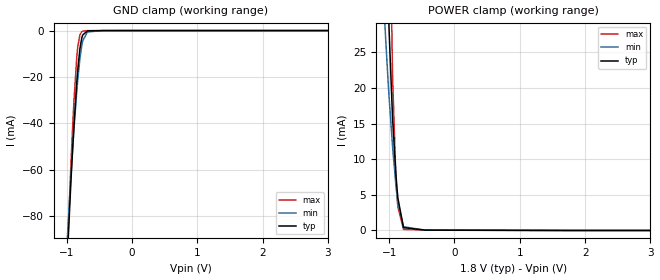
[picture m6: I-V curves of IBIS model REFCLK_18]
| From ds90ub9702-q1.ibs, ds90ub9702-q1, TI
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|   REFCLK_18 model
[Model]   REFCLK_18
Model_type   Input
Vinl = 0.63
Vinh = 1.17
|   typ   min   max
C_comp   1.10571pF   1.21238pF   5pF
[Voltage Range]   1.8   1.71   1.89
[Temperature Range]   27   105   -40
[Power Clamp Reference]   1.8   1.71   1.89
[GND Clamp Reference]   0   0   0
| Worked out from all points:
|   GND clamp passes 1 mA (typ) near -0.72 V on its own axis
|   POWER clamp passes 1 mA (typ) near -0.79 V on its own axis
[GND Clamp]
|   Voltage   I(typ)   I(min)   I(max)
-1.8V     -695.2mA   -622.8mA   -751.1mA
-1.001V   -105mA     -95.31mA   -104mA
-936mV    -66.2mA    -63.73mA   -59.18mA
-909mV    -51.71mA   -51.7mA    -42.45mA
-887.4mV  -40.99mA   -42.6mA    -30.38mA
-844.2mV  -22.35mA   -26.22mA   -11.45mA
-828mV    -16.57mA   -20.87mA   -6.784mA
-795.6mV  -7.686mA   -11.94mA   -1.813mA
-757.8mV  -2.294mA   -5.08mA    -324.2uA
-682.2mV  -140uA     -594.6uA   -25.34uA
-444.6mV  -9.322uA   -8.429uA   -11.13uA
3.6V      0A         0A         0A
[POWER Clamp]
|   Voltage   I(typ)   I(min)   I(max)
-1.8V     913.3mA    660mA      1.143A
-1.076V   62.45mA    31.29mA    126.5mA
-1.055V   49.98mA    27.29mA    103mA
-1.012V   31.67mA    20.38mA    61.71mA
-1.001V   28.28mA    18.81mA    53.01mA
-946.8mV  15.76mA    11.75mA    21.59mA
-898.2mV  8.22mA     6.549mA    7.96mA
-876.6mV  5.652mA    4.69mA     4.554mA
-865.8mV  4.556mA    3.885mA    3.297mA
-779.4mV  399.7uA    531uA      153.8uA
-444.6mV  47.04uA    39.07uA    58.46uA
3.6V      0A         0A         0A
